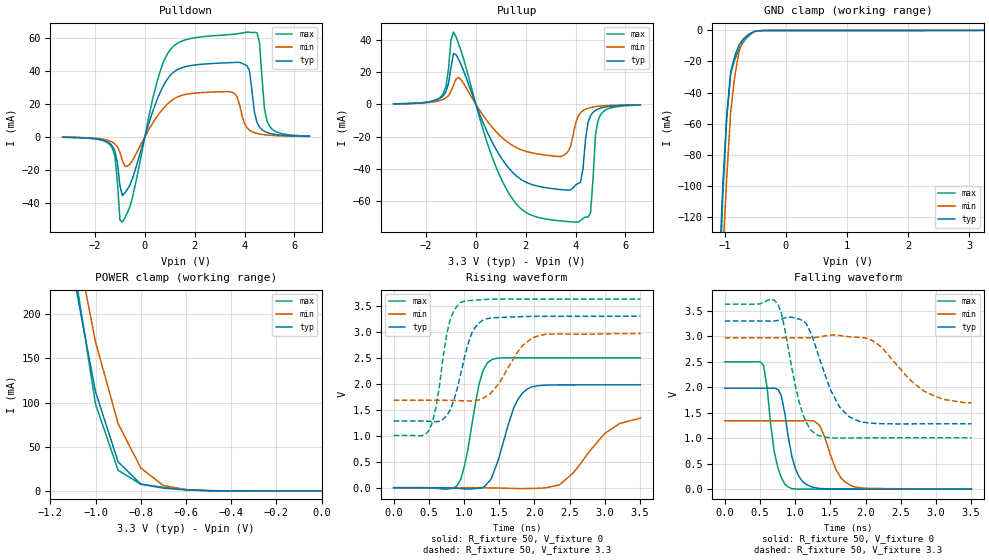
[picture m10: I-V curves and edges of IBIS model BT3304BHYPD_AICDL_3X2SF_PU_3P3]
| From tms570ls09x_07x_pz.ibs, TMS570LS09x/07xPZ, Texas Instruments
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|   Model Cell BT3304BHYPD_AICDL_3X2SF_PU_3P3
|BT3304BHYPD_AICDL_3X2SF_PU_3P3
[Model]   BT3304BHYPD_AICDL_3X2SF_PU_3P3
Model_type   I/O
Polarity   Non-Inverting
Enable   Active-Low
Vinl =  1.15
Vinh =  1.55
Cref =  15.0001pF
Rref =  101.0000M
Vref =  0V
Vmeas =  1.65
C_comp   1.2p   1.2p   1.2p
[Model Spec]
Vinl   1.15   1.02   1.28
Vinh   1.55   1.45   1.65
[Temperature Range]   25   155   -40
[Voltage Range]   3.3   2.97   3.63
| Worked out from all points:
|   slope of the pulldown table from 0 to 0.495 V, typ, clamps not added: 22 ohm
|   slope of the pullup table from 0 to 0.495 V, typ, clamps not added: 26.9 ohm
|   GND clamp passes 1 mA (typ) near -0.53 V on its own axis
|   POWER clamp passes 1 mA (typ) near -0.59 V on its own axis
|   rising waveform, R_fixture 50, V_fixture 0: 20-80 % time 273ps typ, 493ps min, 197ps max; typ from 0.001 V to 1.98 V
|   rising waveform, R_fixture 50, V_fixture 3.3: 20-80 % time 234ps typ, 362ps min, 181ps max; typ from 1.28 V to 3.3 V
|   falling waveform, R_fixture 50, V_fixture 0: 20-80 % time 166ps typ, 226ps min, 141ps max; typ from 1.98 V to 0.001 V
|   falling waveform, R_fixture 50, V_fixture 3.3: 20-80 % time 335ps typ, 534ps min, 238ps max; typ from 3.3 V to 1.28 V
[POWER_clamp]
|   voltage   I(typ)   I(min)   I(max)
-3.3V     4.054A     4.63A      4.887A
-1.1V     248.3mA    301mA      262.8mA
-1.067V   202.9mA    256.9mA    208mA
-1.033V   157.6mA    212.7mA    153.2mA
-1V       112.2mA    168.6mA    98.37mA
-900mV    32.94mA    76.25mA    23.31mA
-800mV    7.767mA    25.97mA    7.563mA
-700mV    3.087mA    6.069mA    4.066mA
-600mV    1.133mA    1.556mA    1.49mA
-500mV    225uA      392.2uA    256.9uA
0V        441.5pA    6.157nA    415.4pA
[Pulldown]
|   voltage   I(typ)   I(min)   I(max)
-3.3V     -289uA     -253.9uA   -287.1uA
-1.4V     -4mA       -2.489mA   -4.76mA
-1.2V     -8.69mA    -4.261mA   -12.05mA
-1V       -29.49mA   -9.376mA   -50.19mA
-900mV    -35.6mA    -14.42mA   -51.6mA
1V        36.78mA    21.07mA    52.28mA
3.5V      44.86mA    26.91mA    61.93mA
4.1V      42.98mA    5.456mA    63.29mA
4.6V      5.887mA    1.718mA    56.92mA
4.8V      3.323mA    1.257mA    16.92mA
5V        2.171mA    957.9uA    6.458mA
6.6V      331.3uA    239.5uA    466.8uA
[Pullup]
|   voltage   I(typ)   I(min)   I(max)
-3.3V     325.3uA    297.6uA    301.6uA
-1.4V     4.042mA    2.556mA    4.795mA
-1.2V     7.932mA    4.062mA    11.12mA
-900mV    31.45mA    11.76mA    44.76mA
1.4V      -40.91mA   -24.77mA   -56.99mA
3.4V      -52.76mA   -32.29mA   -72.18mA
4V        -50.08mA   -11.8mA    -72.98mA
4.2V      -48.37mA   -5.201mA   -71.98mA
4.6V      -7.019mA   -1.989mA   -67.23mA
4.8V      -3.708mA   -1.414mA   -19.03mA
5V        -2.349mA   -1.055mA   -6.475mA
6.6V      -340.9uA   -258.1uA   -448.7uA
[GND_clamp]
|   voltage   I(typ)   I(min)   I(max)
-3.3V     -3.25A     -2.875A    -4.945A
-1.1V     -166.9mA   -205.1mA   -187mA
-1.033V   -102.8mA   -146.7mA   -110.1mA
-966.7mV  -55.98mA   -95.7mA    -57.04mA
-900mV    -26.57mA   -52.04mA   -27.83mA
-833.3mV  -16.54mA   -29.29mA   -18.85mA
-766.7mV  -9.604mA   -13.93mA   -12.19mA
-700mV    -5.772mA   -5.956mA   -7.84mA
-566.7mV  -1.652mA   -1.675mA   -2.192mA
-500mV    -488.4uA   -640.8uA   -598.2uA
-366.7mV  -105uA     -106.2uA   -156.1uA
3.233V    -4.592uA   15.81uA    -37.39uA
[Ramp]
| variable   typ   min   max
dV/dt_f   1.258666/0.3441389n  0.8100911/0.5626007n   1.636857/0.2459206n
dV/dt_r   1.202753/0.2763316n  0.8164284/0.5017067n   1.51672/0.1984257n
R_load = 50
[Rising Waveform]
R_fixture = 50
V_fixture = 0
V_fixture_min = 0
V_fixture_max = 0
|   time   V(typ)   V(min)   V(max)
0s        1.173mV    961uV      1.367mV
904ps     -11.51mV   1.165mV    44.81mV
1.008ns   -21.33mV   1.212mV    434.4mV
1.208ns   -7.384mV   -218.3uV   1.966V
1.408ns   252mV      -3.972mV   2.474V
1.708ns   1.549V     -12.96mV   2.501V
1.904ns   1.906V     -14.2mV    2.5V
2.356ns   1.979V     56.36mV    2.499V
3.004ns   1.98V      1.052V     2.499V
3.504ns   1.98V      1.343V     2.499V
[Rising Waveform]
R_fixture = 50
V_fixture = 3.3
V_fixture_min = 2.97
V_fixture_max = 3.63
|   time   V(typ)   V(min)   V(max)
0s        1.283V     1.684V     1.009V
504ps     1.278V     1.684V     1.107V
604ps     1.273V     1.684V     1.565V
756ps     1.394V     1.683V     2.969V
804ps     1.494V     1.682V     3.244V
956ps     2.208V     1.675V     3.57V
1.108ns   2.971V     1.67V      3.605V
1.284ns   3.241V     1.735V     3.621V
1.968ns   3.298V     2.884V     3.63V
3.504ns   3.3V       2.969V     3.63V
[Falling Waveform]
R_fixture = 50
V_fixture = 0
V_fixture_min = 0
V_fixture_max = 0
|   time   V(typ)   V(min)   V(max)
0s        1.981V     1.343V     2.499V
552ps     1.981V     1.343V     2.427V
704ps     1.983V     1.343V     738.5mV
804ps     1.837V     1.343V     231.1mV
904ps     1.014V     1.343V     41.98mV
1.056ns   244.9mV    1.343V     1.764mV
1.256ns   37.89mV    1.34V      2.028mV
1.656ns   3.649mV    212.3mV    1.835mV
1.836ns   2.472mV    48.86mV    1.818mV
3.504ns   1.471mV    1.502mV    1.394mV
[Falling Waveform]
R_fixture = 50
V_fixture = 3.3
V_fixture_min = 2.97
V_fixture_max = 3.63
|   time   V(typ)   V(min)   V(max)
0s        3.3V       2.97V      3.63V
756ps     3.311V     2.97V      3.635V
804ps     3.333V     2.97V      3.456V
1.108ns   3.312V     2.97V      1.478V
1.308ns   2.728V     2.979V     1.065V
1.508ns   1.935V     3.023V     1.01V
1.772ns   1.416V     2.99V      1.005V
2.16ns    1.289V     2.857V     1.009V
2.876ns   1.283V     1.891V     1.009V
3.504ns   1.284V     1.695V     1.01V
